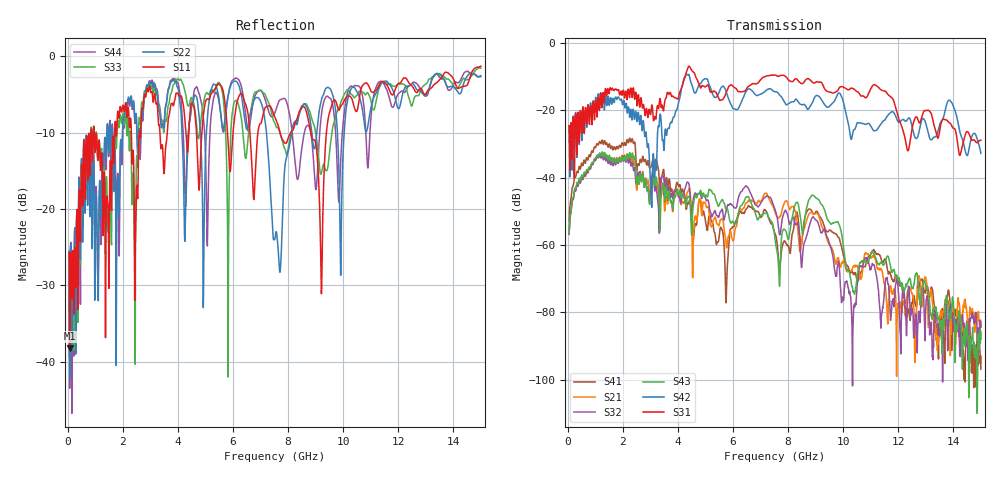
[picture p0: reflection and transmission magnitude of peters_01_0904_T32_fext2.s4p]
# MHZ S RI R 50.00
! FREQ  S11  S12  S13  S14
!  S21  S22  S23  S24
!  S31  S32  S33  S34
!  S41  S42  S43  S44
!  REAL  IMAG  REAL  IMAG  REAL  IMAG  REAL  IMAG
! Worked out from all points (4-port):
!   1496 points, 50 MHz to 15 GHz, reference 50 ohm
!   strongest paths, dB at 50 MHz, 3.79 GHz, 7.53 GHz, 11.27 GHz, 15 GHz:
!     S31: -24.6, -15.9, -9.6, -13.1, -28.9
!     S42: -24.8, -23.4, -14.5, -25.3, -32.8
!     S43: -56.6, -48.1, -58.5, -65.8, -88.0
!     S32: -56.8, -45.4, -49.5, -73.0, -84.5
!     S21: -56.7, -48.8, -50.3, -67.1, -84.1
!     S41: -52.9, -44.1, -56.6, -62.7, -96.9
!   lowest |S11| = -38.3 dB at 70 MHz (marker M1), VSWR 1.02, Z = 50.9 - j0.797 ohm
!   |S11| at or under -10 dB: start of sweep to 847.1 MHz; 964.7 MHz to 1.704 GHz (739.3 MHz wide, 55.4 % of centre); 8.83 GHz to 9.391 GHz (560.9 MHz wide, 6.16 % of centre)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
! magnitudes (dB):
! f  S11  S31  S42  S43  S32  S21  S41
! 50 MHz  -25.7  -24.6  -24.8  -56.6  -56.8  -56.7  -52.9
! 70 MHz  -38.3  -32.9  -33.4  -52.9  -53.3  -53.2  -49.4
! 2.29 GHz  -8.3  -13.4  -19.8  -33.9  -36.3  -34.6  -29.4
! 3.03 GHz  -4.7  -19.6  -43.7  -45.7  -42.4  -45.9  -36.8
! 5.76 GHz  -8.0  -14.6  -14.6  -49.4  -49.8  -60.5  -74.2
! 8.78 GHz  -9.0  -10.9  -19.2  -46.3  -54.2  -50.6  -49.3
! 15 GHz  -1.3  -28.9  -32.8  -88.0  -84.5  -84.1  -96.9
